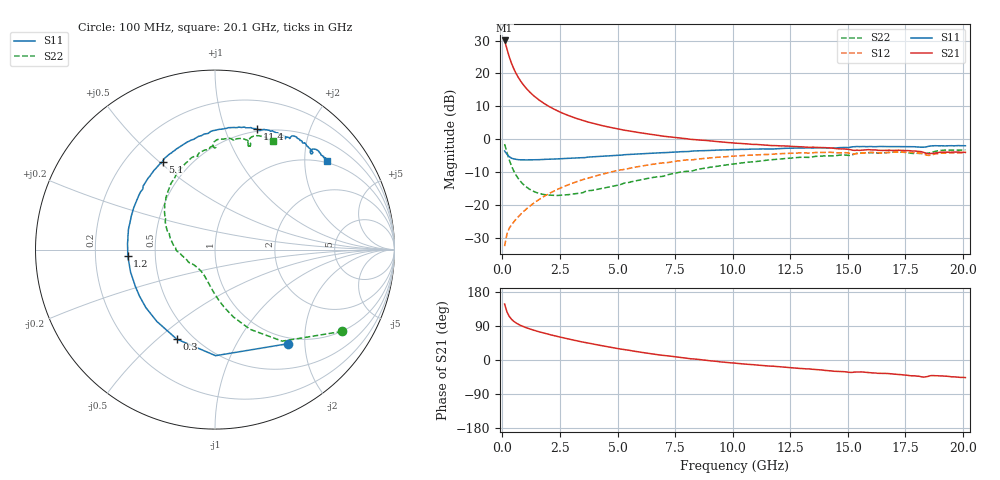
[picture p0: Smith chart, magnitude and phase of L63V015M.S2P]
!  Infineon Technologies AG
! BFR380L3 , PF131585-7, No.6, Th 09.10.01, soldered on pcb-board, measured with PP GSG850
!  Vce=3.0 V,  Ic=15.0 mA
! Common Emitter S-Parameters:  15. November 2001
#  GHz  S  MA  R  50
! f  S11  S21  S12  S22
! GHz  Mag  Ang  Mag  Ang  Mag  Ang  Mag  Ang
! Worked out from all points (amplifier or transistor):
!   201 points, 100 MHz to 20.1 GHz, reference 50 ohm
!   highest |S21| = 30.0 dB at 100 MHz (marker M1)
!   |S21| within 3 dB of that: start of sweep to 218.3 MHz
!   unconditionally stable (mu >= 1): 1.594 GHz to 4.431 GHz
!   at 3.4 GHz: K = 1.02, MAG = 8.3 dB, |S12| = -12.5 dB
!   at 10.1 GHz: K = 0.95, MSG = 2.0 dB, |S12| = -5.1 dB
!   at 20.1 GHz: K = 0.99, MSG = 0.1 dB, |S12| = -4.1 dB
!   S11 on the Smith chart (normalised r, x): 100 MHz: 0.89, -1.67; 300 MHz: 0.41, -0.58; 1.2 GHz: 0.34, -0.03; 5.1 GHz: 0.35, +0.51; 11.4 GHz: 0.48, +1.30; 20.1 GHz: 0.95, +2.56
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0.1  0.6633 -52.2  31.68 147.7  0.02369 63.9  0.8426 -32.7
0.2  0.5911 -89.6  23.58 127.2  0.03612 56.3  0.6329 -53.7
0.3  0.5423 -113.2  17.93 115.3  0.04424 52.5  0.4859 -66.2
0.4  0.5149 -129.0  14.25 107.4  0.04993 52.3  0.3909 -74.6
0.5  0.5027 -140.0  11.74 101.9  0.05555 53.2  0.3274 -80.7
0.6  0.4941 -148.4  9.939 97.7  0.06112 54.3  0.2832 -85.6
0.7  0.4887 -155.2  8.632 94.2  0.06664 55.5  0.2509 -89.9
0.8  0.4856 -160.6  7.613 91.1  0.07239 56.8  0.2262 -93.6
0.9  0.4869 -165.1  6.807 88.5  0.07831 57.7  0.2074 -97.0
1  0.4848 -169.1  6.162 86.1  0.08414 58.6  0.193 -100.1
1.2  0.4874 -175.9  5.176 81.8  0.09655 59.8  0.1724 -105.8
1.6  0.4886 173.5  3.934 74.4  0.1218 60.9  0.1502 -115.9
2.1  0.4964 163.1  3.048 66.4  0.1539 60.4  0.1412 -127.0
2.7  0.5096 152.5  2.421 57.8  0.1925 58.4  0.1422 -139.3
3.5  0.5246 140.5  1.919 47.3  0.2437 54.5  0.1541 -151.7
5.1  0.5712 120.8  1.411 29.2  0.3409 44.6  0.2027 -176.4
6.8  0.6208 103.3  1.139 13.6  0.4298 33.5  0.2701 160.6
10.1  0.6957 78.3  0.8717 -8.3  0.5546 12.0  0.4234 127.7
11.4  0.711 70.6  0.813 -15.2  0.5861 3.6  0.4766 116.1
13.5  0.7353 60.7  0.7566 -24.6  0.623 -8.9  0.5416 99.8
16.8  0.7721 48.2  0.6812 -36.0  0.6297 -25.0  0.6314 78.3
20.1  0.7952 38.4  0.6324 -46.4  0.6224 -38.7  0.6871 61.9
